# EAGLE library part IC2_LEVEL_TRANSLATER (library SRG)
I2C Level Translator PCA9306 Data Sheet Sparkfun breakout board schematic
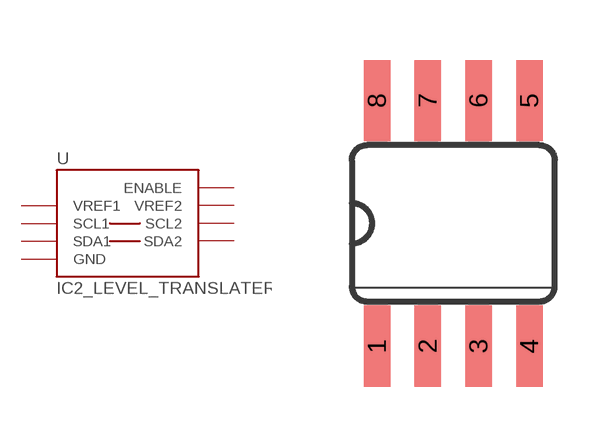
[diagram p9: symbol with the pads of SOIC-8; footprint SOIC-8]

Designator prefix -

## IC2_LEVEL_TRANSLATER  [SOIC-8]
1  VREF1  pwr
2  SCL1
3  SDA1
4  GND  pwr
5  SDA2
6  SCL2
7  VREF2  pwr
8  ENABLE  in

## Footprint SOIC-8 (pad centres in mm)
SOIC-8 Package 0.05" (1.27mm) lead pitch Body 3.8 mm x 4.9 mm
smd 0.66 x 2.032: 1 -1.905,-3.073; 2 -0.635,-3.073; 3 0.635,-3.073; 4 1.905,-3.073; 5 1.905,3.073; 6 0.635,3.073; 7 -0.635,3.073; 8 -1.905,3.073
